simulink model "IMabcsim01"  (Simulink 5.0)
settings: Solver=ode45  StartTime=0.0  StopTime=2  RelTol=1e-3
InitFcn:
  | imparamsim0
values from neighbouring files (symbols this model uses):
  Bm = 0.10    (= 0.1)    [IMabc2.m]    (also in imabcparam.m = 0.01; IMabcrun0.m = 0.01; IMabcrun1.m = 0.001; IMcur0.m = 1e-06)
  gam = 2*pi/3    (= 2.09439510239)    [IMabc2.m]    (also in IMabcf0.m; IMabcf1.m; imabcparam.m; IMabcrun0.m)
  J = 0.02    [imabcparam.m]    (also in IMabcrun0.m; IMabcrun1.m; imdefSIvec1.m = 0.03)
  Lm1 = 2/3*Lm    [IMabcf0.m]    (also in IMabcf1.m; imabcparam.m = 0.0564666666667; IMabcrun0.m = 0.0564666666667; IMabcrun1.m = 0.0564666666667)
  Lrr = [Lr   -Lm/2 -Lm/2    [IMabc2.m]    (also in IMabcf0.m = [Lr   -Lm1/2 -Lm1/2; IMabcf1.m = [Lr   -Lm1/2 -Lm1/2)
  Lss = [Ls   -Lm/2 -Lm/2    [IMabc2.m]    (also in IMabcf0.m = [Ls   -Lm1/2 -Lm1/2; IMabcf1.m = [Ls   -Lm1/2 -Lm1/2)
  nsync = 120*freq0/p    (= 1800)    [imabcparam.m]
  p = cos(beta-alpha)    [abcRwdg.m]    (also in alternator.m = 0:pi/20:2*pi; altwdgs.m = 0:pi/20:2*pi; brushlessdcB.m = 0:pi/100:2*pi; brushlessdcnew.m = 0:pi/100:2*pi)
  R = str2num(get(h,'string'))    [acttrcalc1.m]    (also in IMabc2.m = diag([Rs Rs Rs Rr Rr Rr]); IMabcf0.m = diag([Rs Rs Rs Rr Rr Rr]); IMabcf1.m = diag([Rs Rs Rs Rr Rr Rr]); IMcurf0.m = diag([Rs Rs Rr Rr]))
  Vm = Vll*sqrt(2/3)    [imabcparam.m]
  wo = 2*pi*freq0    [calc0.m]    (also in IMabc2.m = 376.991118431; imabcparam.m = 376.991118431; IMabcrun0.m = 376.991118431; IMabcrun1.m = 376.991118431)
undefined symbols (not defined in the file or in its folder): TL1, TL2
libraries: simulink x9

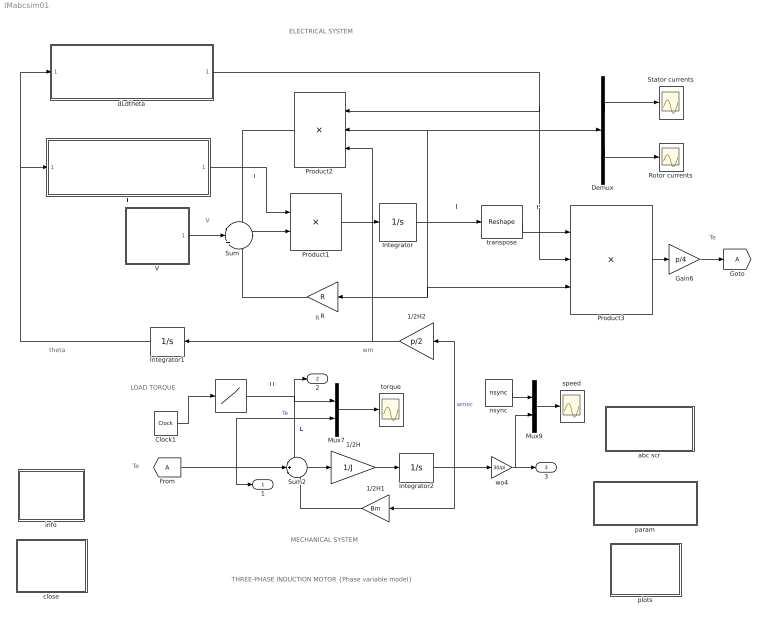
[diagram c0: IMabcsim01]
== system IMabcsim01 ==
  note: I
  note: I'
  note: MECHANICAL SYSTEM
  note: ELECTRICAL SYSTEM
  note: V
  note: wm
  note: theta
  note: THREE-PHASE INDUCTION MOTOR {Phase variable model}
  note: L
  note: Te
  note: TL
  note: Te
  note: LOAD TORQUE
  note: R
  " " : Lookup  InputValues=[0 0.6 0.6 1.4 1.4 2]  OutputValues="[TL1 TL1  TL2 TL2 TL1 TL1]"
  1/2H : Gain  Gain=1/J
  1/2H1 : Gain  Orientation=left  Gain=Bm
  1/2H2 : Gain  Orientation=left  Gain=p/2
  Clock1 : Clock
  Demux : Demux  Outputs=2
  Gain6 : Gain  Gain=p/4  ShowAdditionalParam=on
  Integrator : Integrator  InitialCondition=[0 ;0 ;0; 0 ;0 ;0]
  Integrator1 : Integrator  Orientation=left
  Integrator2 : Integrator  InitialCondition=wo*2/p
  L : Subsystem
  Mux7 : Mux  Inputs=2
  Mux9 : Mux  Inputs=2
  Product1 : Product  Inputs=/*  Multiplication=Matrix(*)
  Product2 : Product  Orientation=left  Inputs=***  Multiplication=Matrix(*)
  Product3 : Product  Inputs=3  Multiplication=Matrix(*)  ShowAdditionalParam=on
  R : Gain  Orientation=left  Gain=R  Multiplication=Matrix(K*u)
  Rotor currents : Scope
  Stator currents : Scope
  Sum : Sum  Inputs=-|+|-
  Sum2 : Sum  Inputs=-+-
  V : Subsystem
  abc scr : Subsystem
  close : Subsystem
  dLdtheta : Subsystem
  info : Subsystem
  nsync : Constant  Value=nsync
  param : Subsystem
  plots : Subsystem
  speed : Scope
  torque : Scope
  transpose : simulink/Math Operations/Reshape  OutputDimensionality=Row vector  OutputDimensions=[1,6]
  wo4 : Gain  Gain=30/pi
  1 : Outport
  2 : Outport  Port=2
  3 : Outport  Port=3
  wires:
  Product1/1 -> Integrator/1
  Integrator/1 -> Product3/3, R/1, transpose/1, Product2/2, Demux/1
  Sum/1 -> Product1/2
  R/1 -> Sum/3
  transpose/1 -> Product3/1
  Demux/1 -> Stator currents/1
  Demux/2 -> Rotor currents/1
  Product2/1 -> Sum/1
  dLdtheta/1(dLdtheta) -> Product2/1, Product3/2
  Product3/1 -> Gain6/1
  Gain6/1 -> [A]
  Sum2/1 -> 1/2H/1
  1/2H/1 -> Integrator2/1
  1/2H1/1 -> Sum2/3
  wo4/1 -> Mux9/2, 3/1
  Mux9/1 -> speed/1
  nsync/1 -> Mux9/1
  Mux7/1 -> torque/1
  " "/1 -> Mux7/1, Sum2/1, 2/1  "TL"
  [A] -> Sum2/2, 1/1, Mux7/2  "Te"
  Integrator2/1 -> wo4/1, 1/2H1/1, 1/2H2/1  "wmec"
  V/1(V) -> Sum/2
  1/2H2/1 -> Integrator1/1, Product2/3
  Integrator1/1 -> dLdtheta/1(theta1), L/1(theta)
  L/1(L) -> Product1/1
  Clock1/1 -> " "/1

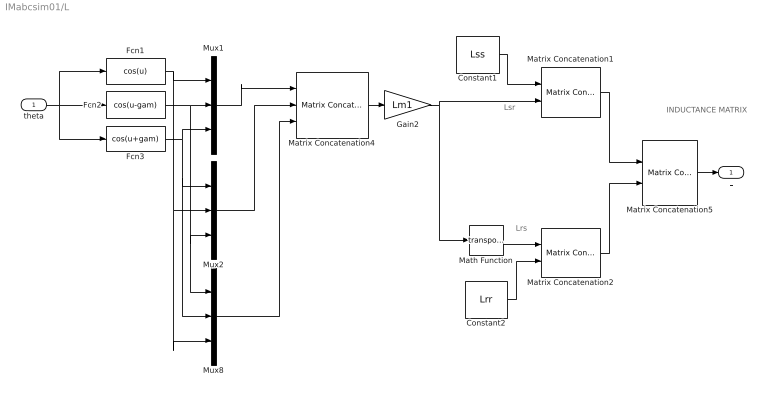
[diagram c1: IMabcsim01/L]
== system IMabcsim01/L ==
  note: INDUCTANCE MATRIX
  note: Lsr
  note: Lrs
  theta : Inport
  Constant1 : Constant  Value=Lss  VectorParams1D=off
  Constant2 : Constant  Value=Lrr  VectorParams1D=off
  Fcn1 : Fcn  Expr=cos(u)
  Fcn2 : Fcn  Expr=cos(u-gam)
  Fcn3 : Fcn  Expr=cos(u+gam)
  Gain2 : Gain  Gain=Lm1
  Math Function : Math  Operator=transpose
  Matrix Concatenation1 : simulink/Math Operations/Matrix Concatenation  numInports=2  catMethod=Horizontal
  Matrix Concatenation2 : simulink/Math Operations/Matrix Concatenation  numInports=2  catMethod=Horizontal
  Matrix Concatenation4 : simulink/Math Operations/Matrix Concatenation  numInports=3  catMethod=Horizontal
  Matrix Concatenation5 : simulink/Math Operations/Matrix Concatenation  numInports=2  catMethod=Vertical
  Mux1 : Mux  Inputs=3
  Mux2 : Mux  Inputs=3
  Mux8 : Mux  Inputs=3
  L : Outport
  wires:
  Matrix Concatenation5/1 -> L/1
  theta/1 -> Fcn3/1, Fcn1/1, Fcn2/1
  Math Function/1 -> Matrix Concatenation2/1
  Gain2/1 -> Matrix Concatenation1/2, Math Function/1
  Mux1/1 -> Matrix Concatenation4/1
  Matrix Concatenation4/1 -> Gain2/1
  Mux8/1 -> Matrix Concatenation4/3
  Mux2/1 -> Matrix Concatenation4/2
  Matrix Concatenation1/1 -> Matrix Concatenation5/1
  Matrix Concatenation2/1 -> Matrix Concatenation5/2
  Constant1/1 -> Matrix Concatenation1/1
  Constant2/1 -> Matrix Concatenation2/2
  Fcn3/1 -> Mux1/3, Mux2/1, Mux8/2
  Fcn2/1 -> Mux1/2, Mux2/3, Mux8/1
  Fcn1/1 -> Mux8/3, Mux2/2, Mux1/1

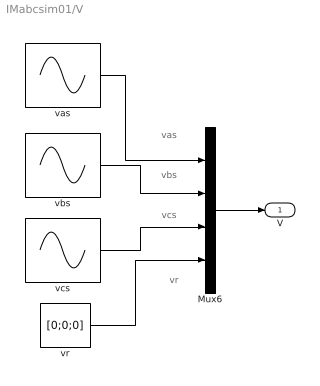
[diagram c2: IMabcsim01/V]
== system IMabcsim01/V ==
  note: vas
  note: vbs
  note: vcs
  note: vr
  Mux6 : Mux
  vas : Sin  Amplitude=Vm  Frequency=wo  Phase=pi/2  SampleTime=0
  vbs : Sin  Amplitude=Vm  Frequency=wo  Phase=pi/2-gam  SampleTime=0
  vcs : Sin  Amplitude=Vm  Frequency=wo  Phase=pi/2+gam  SampleTime=0
  vr : Constant  Value=[0;0;0]  VectorParams1D=off
  V : Outport
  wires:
  Mux6/1 -> V/1
  vr/1 -> Mux6/4
  vcs/1 -> Mux6/3
  vbs/1 -> Mux6/2
  vas/1 -> Mux6/1

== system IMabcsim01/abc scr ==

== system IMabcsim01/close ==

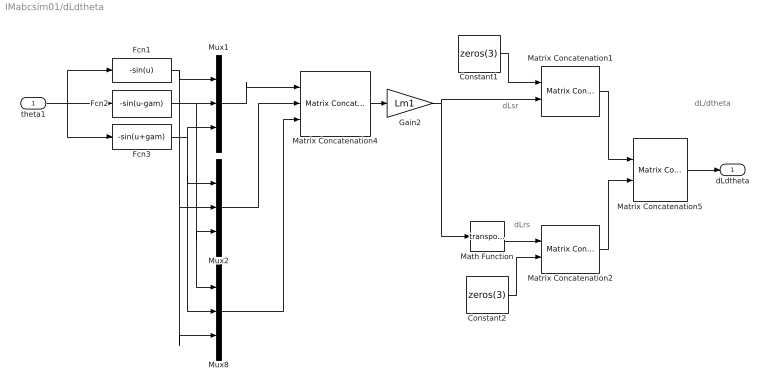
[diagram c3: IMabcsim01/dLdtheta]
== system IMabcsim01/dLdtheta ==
  note: dL/dtheta
  note: dLsr
  note: dLrs
  theta1 : Inport
  Constant1 : Constant  Value=zeros(3)  VectorParams1D=off
  Constant2 : Constant  Value=zeros(3)  VectorParams1D=off
  Fcn1 : Fcn  Expr=-sin(u)
  Fcn2 : Fcn  Expr=-sin(u-gam)
  Fcn3 : Fcn  Expr=-sin(u+gam)
  Gain2 : Gain  Gain=Lm1
  Math Function : Math  Operator=transpose
  Matrix Concatenation1 : simulink/Math Operations/Matrix Concatenation  numInports=2  catMethod=Horizontal
  Matrix Concatenation2 : simulink/Math Operations/Matrix Concatenation  numInports=2  catMethod=Horizontal
  Matrix Concatenation4 : simulink/Math Operations/Matrix Concatenation  numInports=3  catMethod=Horizontal
  Matrix Concatenation5 : simulink/Math Operations/Matrix Concatenation  numInports=2  catMethod=Vertical
  Mux1 : Mux  Inputs=3
  Mux2 : Mux  Inputs=3
  Mux8 : Mux  Inputs=3
  dLdtheta : Outport
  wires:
  theta1/1 -> Fcn1/1, Fcn2/1, Fcn3/1
  Math Function/1 -> Matrix Concatenation2/1
  Gain2/1 -> Matrix Concatenation1/2, Math Function/1
  Mux1/1 -> Matrix Concatenation4/1
  Matrix Concatenation4/1 -> Gain2/1
  Mux8/1 -> Matrix Concatenation4/3
  Mux2/1 -> Matrix Concatenation4/2
  Matrix Concatenation1/1 -> Matrix Concatenation5/1
  Matrix Concatenation2/1 -> Matrix Concatenation5/2
  Constant1/1 -> Matrix Concatenation1/1
  Constant2/1 -> Matrix Concatenation2/2
  Fcn3/1 -> Mux1/3, Mux2/1, Mux8/2
  Fcn2/1 -> Mux1/2, Mux2/3, Mux8/1
  Fcn1/1 -> Mux8/3, Mux2/2, Mux1/1
  Matrix Concatenation5/1 -> dLdtheta/1

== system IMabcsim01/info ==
  note: INDUCTION MOTOR RUNNING UNDER PULSED LOADS (Phase variable model) SI units
  note: The three-phase motor is running in steady state at a specified load when a pulsating torque load is appled. The machine dynamic equations are based on a matrix equivalent formulation in Simulink in which the state variables are the phase variables, namely the stator currents ias, ibs, ics and the rotor currents iar, ibr, icr; the the rotor speed wm; and the angular displacement between stator ax_axis and rotor ar_axis. The parameters describing the electromechanical system are expressed in SI units and may be modified by accessing a data file obtained by clicking the PARAMETERS block. The torque developed, the speed, and the stator current are observed on the scopes . The torque-speed dynamic characteristics can then be obtained after double clicking the PLOTS block. To run the identical operation of this motor now formulated in a Matlab script file, run > or double click block. To run the identical operation in the space variable model using DQ, access the Simulink model file >.

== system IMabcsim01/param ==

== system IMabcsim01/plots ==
